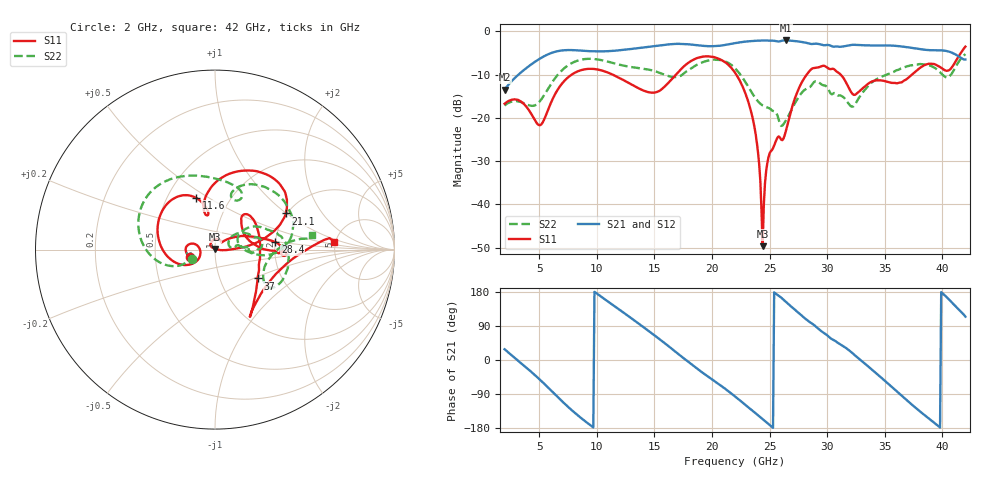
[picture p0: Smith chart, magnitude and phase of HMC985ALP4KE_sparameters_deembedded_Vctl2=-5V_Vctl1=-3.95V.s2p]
!s2p File: Measurements: S11, S21, S12, S22
# GHz S dB R 50.0
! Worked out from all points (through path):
!   401 points, 2 GHz to 42 GHz, reference 50 ohm
!   highest |S21| = -2.11 dB at 26.4 GHz (marker M1); lowest = -13.5 dB at 2 GHz (marker M2)
!   lowest |S11| = -49.7 dB at 24.4 GHz (marker M3), VSWR 1.01, Z = 50 + j0.329 ohm
!   |S11| at or under -10 dB: start of sweep to 7.831 GHz; 22.11 GHz to 28.22 GHz (6.114 GHz wide, 24.3 % of centre); 31.17 GHz to 37.37 GHz (6.199 GHz wide, 18.1 % of centre)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
!   |S22| runs from -21.9 to -5.3 dB; largest |S21 - S12| = 0.00088
!   S11 on the Smith chart (normalised r, x): 2 GHz: 0.75, -0.07; 11.6 GHz: 0.70, +0.44; 21.1 GHz: 1.97, +0.99; 28.4 GHz: 2.00, +0.19; 37 GHz: 1.51, -0.53; 42 GHz: 4.86, +0.76
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2  -16.74 -162.8  -13.50 28.3  -13.50 28.3  -17.15 -157.3
5.1  -21.67 -169.4  -6.25 -52.9  -6.26 -52.9  -16.03 -158.8
6.3  -14.93 -151.4  -4.79 -88.3  -4.79 -88.3  -11.12 -161.5
8.7  -8.93 149.9  -4.47 -154.7  -4.47 -154.6  -6.52 151.3
11.6  -10.29 109.9  -4.47 140.8  -4.48 140.8  -7.46 103.7
13.6  -13.12 100.7  -3.88 96.9  -3.88 96.9  -8.49 76.2
15.4  -13.82 105.3  -3.28 56.1  -3.28 56.1  -9.53 63.0
17.9  -7.36 79.6  -2.99 -3.9  -2.99 -3.9  -9.07 72.0
21.1  -7.08 27.1  -3.17 -74.8  -3.17 -74.8  -6.90 15.9
22  -9.54 16.6  -2.74 -96.1  -2.74 -96.1  -8.53 0.6
23.6  -20.91 0.6  -2.22 -135.9  -2.22 -135.9  -14.76 -3.4
24.4  -49.65 88.3  -2.13 -156.1  -2.13 -156.0  -17.13 7.7
25  -28.22 131.6  -2.16 -171.3  -2.16 -171.3  -17.80 10.9
26.4  -23.20 44.0  -2.11 153.9  -2.11 154.0  -20.68 32.7
28.4  -9.40 7.1  -2.80 101.9  -2.80 102.0  -13.01 18.2
28.7  -8.60 1.9  -2.93 95.8  -2.94 95.8  -12.26 16.5
30.7  -8.99 -3.3  -3.52 50.4  -3.52 50.4  -14.33 2.6
32.5  -14.52 34.3  -3.14 9.9  -3.14 9.9  -16.58 29.5
35.4  -11.76 18.1  -3.27 -65.5  -3.27 -65.4  -9.78 19.1
37  -10.84 -34.0  -3.69 -108.5  -3.70 -108.5  -8.05 4.7
39.8  -8.25 -56.3  -4.39 -178.2  -4.39 -178.1  -9.46 -34.2
42  -3.54 3.8  -6.50 114.4  -6.50 114.4  -5.27 8.5
